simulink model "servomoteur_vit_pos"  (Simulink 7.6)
settings: Solver=ode14x  StartTime=0.0  StopTime=80  FixedStep=0.01  MaxStep=0.01  MinStep=0.001  RelTol=1e-3
InitFcn:
  | close all
StopFcn:
  | load servo_pos_vit.mat
  | plotyy(x(1,:),x(2,:),x(1,:),x(3,:)), grid
  | title('Position et vitesse angulaires')
  | xlabel('temps')
  | figure
  | plot(x(1,:),x(4,:))
  | title('vitesse en sortie w du bloc moteur'), grid
  | xlabel('temps')
  | delete *.mat
libraries: fl_lib x8, nesl_utility x4, elec_lib x2

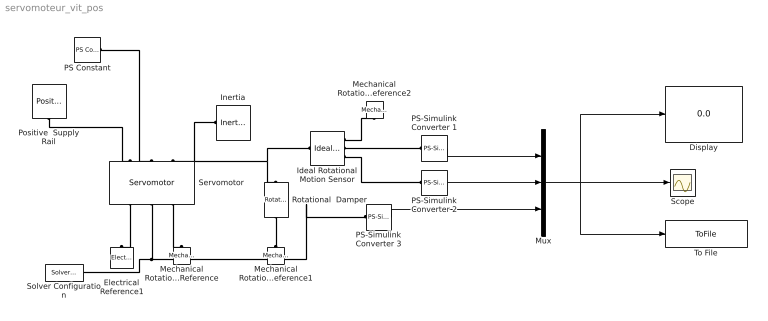
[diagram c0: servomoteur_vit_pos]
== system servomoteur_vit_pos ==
  Display : Display
  Electrical Reference1 : fl_lib/Electrical/Electrical Elements/Electrical Reference  DialogController=NetworkEngine.DynNeDlgSource  SystemSampleTime=-1  i_Log=off  LocalVarNames=|i  LocalVarDescs=|i  LocalVarLogging=[]
  Ideal Rotational Motion Sensor : fl_lib/Mechanical/Mechanical Sensors/Ideal Rotational Motion Sensor  DialogController=NetworkEngine.DynNeDlgSource  SystemSampleTime=-1  offset=0 rad  w_Log=off  t_Log=off  phi_Log=off  LocalVarNames=|w|t|phi  LocalVarDescs=|w|t|phi  LocalVarLogging=[]
  Inertia : fl_lib/Mechanical/Rotational Elements/Inertia  DialogController=NetworkEngine.DynNeDlgSource  SystemSampleTime=-1  inertia=0.01 kg*m^2  initial_velocity=0 rad/s  t_Log=off  LocalVarNames=|t  LocalVarDescs=|t  LocalVarLogging=0
  Mechanical Rotational Reference : fl_lib/Mechanical/Rotational Elements/Mechanical Rotational Reference  DialogController=NetworkEngine.DynNeDlgSource  SystemSampleTime=-1  t_Log=off  LocalVarNames=|t  LocalVarDescs=|t  LocalVarLogging=[]
  Mechanical Rotational Reference1 : fl_lib/Mechanical/Rotational Elements/Mechanical Rotational Reference  DialogController=NetworkEngine.DynNeDlgSource  SystemSampleTime=-1  t_Log=off  LocalVarNames=|t  LocalVarDescs=|t  LocalVarLogging=[]
  Mechanical Rotational Reference2 : fl_lib/Mechanical/Rotational Elements/Mechanical Rotational Reference  DialogController=NetworkEngine.DynNeDlgSource  SystemSampleTime=-1  t_Log=off  LocalVarNames=|t  LocalVarDescs=|t  LocalVarLogging=[]
  Mux : Mux  Inputs=3
  PS Constant : fl_lib/Physical Signals/Sources/PS Constant  DialogController=NetworkEngine.DynNeDlgSource  SystemSampleTime=-1  constant=5  LocalVarLogging=[]
  PS-Simulink Converter 1 : nesl_utility/PS-Simulink Converter  DialogController=NetworkEngine.DynNeUtilDlgSource  SystemSampleTime=-1  PhysicalDomain=network_engine_domain  LeftPortType=input  RightPortType=output  SubClassName=ps_output  Unit=rad/s  AffineConversion=off
  PS-Simulink Converter 2 : nesl_utility/PS-Simulink Converter  DialogController=NetworkEngine.DynNeUtilDlgSource  SystemSampleTime=-1  PhysicalDomain=network_engine_domain  LeftPortType=input  RightPortType=output  SubClassName=ps_output  Unit=rad  AffineConversion=off
  PS-Simulink Converter 3 : nesl_utility/PS-Simulink Converter  DialogController=NetworkEngine.DynNeUtilDlgSource  SystemSampleTime=-1  PhysicalDomain=network_engine_domain  LeftPortType=input  RightPortType=output  SubClassName=ps_output  Unit=rad/s  AffineConversion=off
  Positive  Supply Rail : elec_lib/Sources/Positive Supply Rail  DialogController=NetworkEngine.DynNeDlgSource  SystemSampleTime=-1  v0=12 V  current_Log=off  voltage_Log=off  power_Log=off  LocalVarNames=|current|voltage|power  LocalVarDescs=|Current (A)|Voltage (V)|Power (W)  LocalVarLogging=[0 0 0]
  Rotational  Damper : fl_lib/Mechanical/Rotational Elements/Rotational Damper  DialogController=NetworkEngine.DynNeDlgSource  SystemSampleTime=-1  D=0.001 N*m/(rad/s)  t_Log=off  w_Log=off  LocalVarNames=|t|w  LocalVarDescs=|t|w  LocalVarLogging=[0 0]
  Scope : Scope
  Servomotor : elec_lib/Actuators & Drivers/Rotational Actuators/Servomotor  DialogController=NetworkEngine.DynNeDlgSource  SystemSampleTime=-1  w_t="[0  3.75e+03  7.5e+03  8e+03 ] rpm"  T_t=[0.09 0.08 0.07 0 ] N*m  Tc=0.02 s  eff=100  w_eff=3.75e+3 rpm  T_eff=0.08 N*m  Pbase=0 W  Res=3.5 Ohm  J=5e-06 kg*m^2  lam=1e-05 N*m/(rad/s)  speed0=0 rpm  LocalVarLogging=[]
  Solver Configuration : nesl_utility/Solver Configuration  DialogController=NetworkEngine.DynNeUtilDlgSource  SystemSampleTime=-1  PhysicalDomain=network_engine_domain  LeftPortType=input  RightPortType=generic  SubClassName=solver  Accelerate=off  Profile=off  ResidualTolerance=1e-1  MaxNonlinIter=12  MaxModeIter=2  DoFixedCost=on  UseLocalSampling=off  DoDC=off  LinearAlgebra=Sparse  LocalSolverSampleTime=.001  LocalSolverChoice=NE_BACKWARD_EULER_ADVANCER  UseLocalSolver=off
  To File : ToFile  Filename=servo_pos_vit.mat  MatrixName=x
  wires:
  PS-Simulink Converter 1/1 -> Mux/1
  PS-Simulink Converter 2/1 -> Mux/2
  PS-Simulink Converter 3/1 -> Mux/3
  Mux/1 -> Scope/1, To File/1, Display/1
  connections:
  Servomotor/LConn3 -- Ideal Rotational Motion Sensor/LConn1 -- Rotational  Damper/LConn1 -- Inertia/LConn1
  Servomotor/RConn3 -- Mechanical Rotational Reference/LConn1
  Ideal Rotational Motion Sensor/RConn1 -- Mechanical Rotational Reference2/LConn1
  Ideal Rotational Motion Sensor/RConn2 -- PS-Simulink Converter 1/LConn1
  Ideal Rotational Motion Sensor/RConn3 -- PS-Simulink Converter 2/LConn1
  Servomotor/RConn2 -- PS-Simulink Converter 3/LConn1 -- Solver Configuration/RConn1
  PS Constant/RConn1 -- Servomotor/LConn2
  Positive  Supply Rail/RConn1 -- Servomotor/LConn1
  Servomotor/RConn1 -- Electrical Reference1/LConn1
  Rotational  Damper/RConn1 -- Mechanical Rotational Reference1/LConn1
